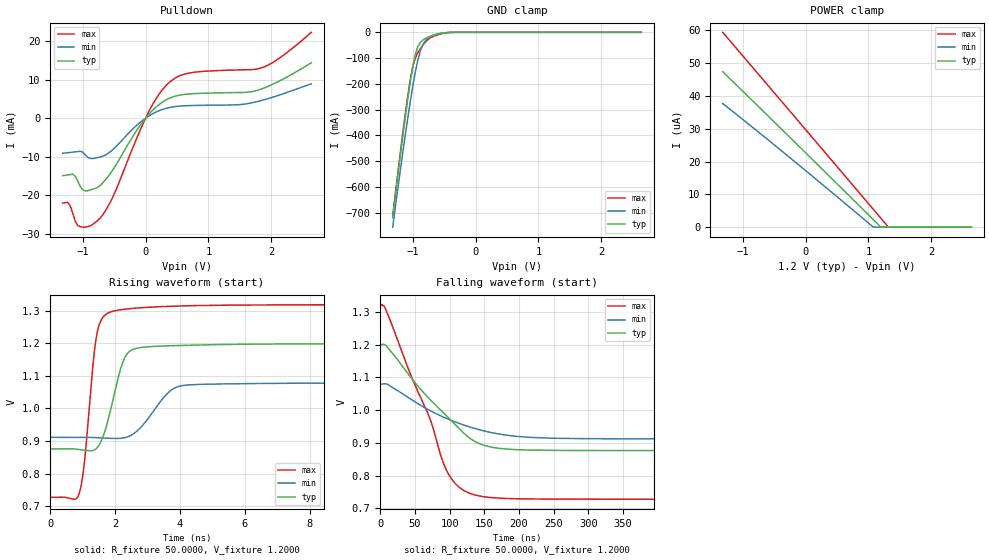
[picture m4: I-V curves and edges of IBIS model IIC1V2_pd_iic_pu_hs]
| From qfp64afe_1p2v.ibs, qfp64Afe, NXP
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[Model] IIC1V2_pd_iic_pu_hs
|   Model IIC1V2_pd_iic_pu_hs
| This model was characterised for following simulation conditions:
| External (pad) voltage:
|   - Typ: 1.2V,   - Min: 1.08V,   - Max: 1.32V
| Library cells for typ/min/max conditions are connected as defined below:
|  IO - External Pad
|  A - Core Input
|  EN - Output Buffer Enable
|  BOOST - vdde
|  ECS - vdd
|  EGP - gnd
|  ENZI - vdd
|  EPD - vdd
|  EPUN - vdd
|  SSEL - vdd
|  ZI - NC
|  ZIF - NC
|  gnd - gnd
|  gnde - gnde
|  vdd - vdd
|  vdde - vdde
| All other pins connected to ground
Model_type I/O_open_drain
Polarity   Non-Inverting
Enable   Active-Low
Vinl =   0.5400V
Vinh =   1.2600V
Vmeas =  0.9000V
Cref =   0.0F
Rref =   1.0000k
Vref =   1.2000V
C_comp   3.6164pF   3.4768pF   3.7417pF
|C_comp_pullup   0.9402pF   0.8991pF   0.9548pF
|C_comp_pulldown   2.3240pF   2.4771pF   2.1787pF
[Model Spec]
| variable   typ   min   max
Vinh   0.3600V   0.3240V   0.3960V
Vinl   0.8400V   0.7560V   0.9240V
Vmeas   0.6000V   0.5400V   0.6600V
Vref   1.2000V   1.0800V   1.3200V
Cref   0.0F   0.0F   0.0F
Rref   1.0000k   1.0000k   1.0000k
[Temperature Range]   25.0000   0.1250k   -40.0000
[Voltage Range]   1.2000V   1.0800V   1.3200V
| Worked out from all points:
|   slope of the pulldown table from 0 to 0.18 V, typ, clamps not added: 58.3 ohm
|   GND clamp passes 1 mA (typ) near -0.45 V on its own axis
|   rising waveform, R_fixture 50.0000, V_fixture 1.2000: 20-80 % time 495ps typ, 789ps min, 329ps max; typ from 0.876 V to 1.2 V
|   falling waveform, R_fixture 50.0000, V_fixture 1.2000: 20-80 % time 83.3ns typ, 98.9ns min, 62.6ns max; typ from 1.2 V to 0.876 V
[Pulldown]
|Voltage   I(typ)   I(min)   I(max)
-1.32V    -14.96mA   -9.099mA   -22.09mA
-1.24V    -14.75mA   -8.982mA   -21.89mA
-1.16V    -14.56mA   -8.83mA    -24.7mA
-1.04V    -17.82mA   -8.609mA   -28.21mA
-920mV    -18.88mA   -10.21mA   -28.21mA
-720mV    -17.44mA   -10.07mA   -25.94mA
-520mV    -13.41mA   -8.157mA   -20.44mA
80mV      1.521mA    840uA      2.628mA
440mV     5.569mA    2.951mA    10.1mA
760mV     6.377mA    3.307mA    11.92mA
1.84V     7.555mA    4.581mA    13.06mA
2.64V     14.41mA    8.944mA    22.34mA
[GND_clamp]
|Voltage   I(typ)   I(min)   I(max)
-1.32V    -720.7mA   -756.5mA   -713.8mA
-1.12V    -330.9mA   -399.5mA   -316.8mA
-1.04V    -192.4mA   -269.2mA   -184.4mA
-1V       -133.6mA   -209.3mA   -133.5mA
-960mV    -86.74mA   -154.7mA   -99.46mA
-920mV    -55.69mA   -108.2mA   -79.02mA
-880mV    -39.02mA   -72.35mA   -63.71mA
-840mV    -29.9mA    -48mA      -50.26mA
-760mV    -18.93mA   -23.39mA   -28.32mA
-640mV    -9.22mA    -8.628mA   -12.73mA
-400mV    -335.3uA   -402.3uA   -442.6uA
2.64V     0A         0A         0A
[POWER_clamp]
|Voltage   I(typ)   I(min)   I(max)
-1.32V    47.4uA     37.67uA    59.39uA
-280mV    27.94uA    21.65uA    36.04uA
1.08V     2.274uA    0A         5.413uA
1.2V      0A         0A         2.707uA
1.32V     0A         0A         0A
2.64V     0A         0A         0A
[Ramp]
| variable   typ   min   max
dV/dt_r  0.1940/0.4949n   0.1007/0.7889n   0.3552/0.3286n
dV/dt_f  0.1940/83.3009n   0.1007/98.8678n   0.3551/62.6103n
R_load = 50.0000
[Rising Waveform]
R_fixture= 50.0000
V_fixture= 1.2000
V_fixture_min= 1.0800
V_fixture_max= 1.3200
|time   V(typ)   V(min)   V(max)
0s        875.8mV    911.4mV    727.2mV
904.2ps   874mV      911.7mV    743.4mV
1.064ns   871.8mV    911.6mV    845.4mV
1.399ns   875.1mV    910.5mV    1.206V
1.675ns   927.2mV    909.2mV    1.286V
2.169ns   1.121V     908.3mV    1.303V
2.472ns   1.177V     916.8mV    1.306V
3.874ns   1.193V     1.065V     1.314V
6.179ns   1.197V     1.076V     1.318V
1us       1.199V     1.079V     1.319V
[Falling Waveform]
R_fixture= 50.0000
V_fixture= 1.2000
V_fixture_min= 1.0800
V_fixture_max= 1.3200
|time   V(typ)   V(min)   V(max)
0s        1.199V     1.079V     1.319V
6.585ns   1.199V     1.08V      1.314V
39.99ns   1.111V     1.039V     1.128V
68.4ns    1.04V      1.002V     990.8mV
94.85ns   983.9mV    974.9mV    818.9mV
112.4ns   946.3mV    960.2mV    766.5mV
135.4ns   905.6mV    944.2mV    741.2mV
175.8ns   881.9mV    925.2mV    730.3mV
250.5ns   876.8mV    913.9mV    727.8mV
1us       875.9mV    911.5mV    727.2mV
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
